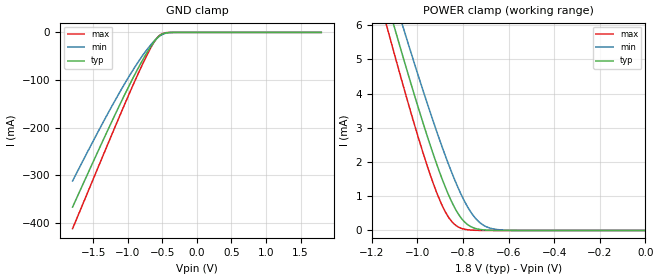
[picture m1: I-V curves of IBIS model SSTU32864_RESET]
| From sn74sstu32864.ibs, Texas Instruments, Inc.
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| NOTE:  The [Diff Pin] section is commented out because the ibischk3 program
|   currently flags it as an Error when it shouldn't
| [Diff Pin]  inv_pin   vdiff   tdelay_typ
|H1   J1   600mV   NA
|A1   A3   580mV   NA
|D1   A3   580mV   NA
|H2   A3   580mV   NA
|B1   A3   580mV   NA
|C1   A3   580mV   NA
|E1   A3   580mV   NA
|F1   A3   580mV   NA
|K1   A3   580mV   NA
|L1   A3   580mV   NA
|M1   A3   580mV   NA
|N1   A3   580mV   NA
|P1   A3   580mV   NA
|R1   A3   580mV   NA
|T1   A3   580mV   NA
|B2   A3   580mV   NA
|C2   A3   580mV   NA
|E2   A3   580mV   NA
|F2   A3   580mV   NA
|K2   A3   580mV   NA
|L2   A3   580mV   NA
|M2   A3   580mV   NA
|N2   A3   580mV   NA
|P2   A3   580mV   NA
|R2   A3   580mV   NA
|T2   A3   580mV   NA
|J2   A3   580mV   NA
[Model]   SSTU32864_RESET
Model_type  Input
Vinl=0.665
Vinh=1.105
| variable   typ   min   max
C_comp   2.18pF   1.72pF   2.37pF
[Temperature Range]   40   85   0
| Ambient temperature   25   70   0
[Voltage range]   1.8   1.7   1.9
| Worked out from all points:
|   GND clamp passes 1 mA (typ) near -0.45 V on its own axis
|   POWER clamp passes 1 mA (typ) near -0.86 V on its own axis
[GND Clamp]
| SSTU32864_RESET
|   Voltage   I(typ)   I(min)   I(max)
-1.8V     -366.3mA   -311.6mA   -411.7mA
-1.34V    -220.5mA   -183.7mA   -251.7mA
-1V       -117.1mA   -96.44mA   -135.4mA
-830mV    -69.48mA   -57.65mA   -80.04mA
-690mV    -34.55mA   -29.9mA    -38.14mA
-605mV    -16.88mA   -15.99mA   -17mA
-535mV    -6.576mA   -7.343mA   -5.649mA
-460mV    -1.429mA   -2.103mA   -934.7uA
-340mV    -49.41uA   -124uA     -18.04uA
1.8V      1.074nA    8.658nA    119.1pA
[POWER Clamp]
| SSTU32864_RESET
|   Voltage   I(typ)   I(min)   I(max)
-1.8V     23.04mA    22.92mA    23.22mA
-1.14V    6.837mA    7.627mA    6.099mA
-1.125V   6.487mA    7.294mA    5.731mA
-1.1V     5.907mA    6.744mA    5.124mA
-1.06V    4.993mA    5.872mA    4.169mA
-970mV    3.024mA    3.974mA    2.152mA
-910mV    1.832mA    2.783mA    1.013mA
-860mV    984.8uA    1.869mA    350.9uA
-815mV    424.9uA    1.147mA    82.3uA
-745mV    57.1uA     352.4uA    5.154uA
-670mV    4.139uA    49.18uA    235.7nA
-16.28fV  1.074nA    8.252nA    134.1pA
